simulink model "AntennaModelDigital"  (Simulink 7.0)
settings: Solver=ode45  StartTime=0.0  StopTime=20  MaxStep=0.01  RelTol=1e-3
libraries: cstblocks x4

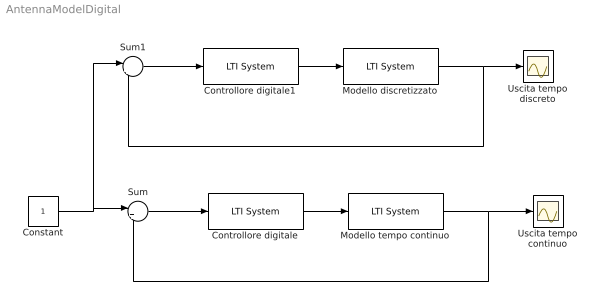
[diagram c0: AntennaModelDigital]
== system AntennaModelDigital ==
  Constant : Constant  OutDataType=sfix(16)  OutScaling=2^0
  Controllore digitale : cstblocks/LTI System  SystemSampleTime=-1  sys=Cd  IC=[]
  Controllore digitale1 : cstblocks/LTI System  SystemSampleTime=-1  sys=Cd  IC=[]
  Modello discretizzato : cstblocks/LTI System  SystemSampleTime=-1  sys=Gd  IC=[]
  Modello tempo continuo : cstblocks/LTI System  SystemSampleTime=-1  sys=G  IC=[]
  Sum : Sum  Inputs=|+-  OutDataType=sfix(16)  OutScaling=2^0
  Sum1 : Sum  Inputs=|+-  OutDataType=sfix(16)  OutScaling=2^0
  Uscita tempo continuo : Scope
  Uscita tempo discreto : Scope
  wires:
  Modello tempo continuo/1 -> Uscita tempo continuo/1, Sum/2
  Sum/1 -> Controllore digitale/1
  Constant/1 -> Sum/1, Sum1/1
  Controllore digitale/1 -> Modello tempo continuo/1
  Modello discretizzato/1 -> Sum1/2, Uscita tempo discreto/1
  Sum1/1 -> Controllore digitale1/1
  Controllore digitale1/1 -> Modello discretizzato/1
